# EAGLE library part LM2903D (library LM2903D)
LM2903DG4, Dual Comparator Open Collector 1.3s 2-kanalers 3, 5, 9, 12, 15, 18, 24, 28V 8-Pin SOIC Source: Datasheet
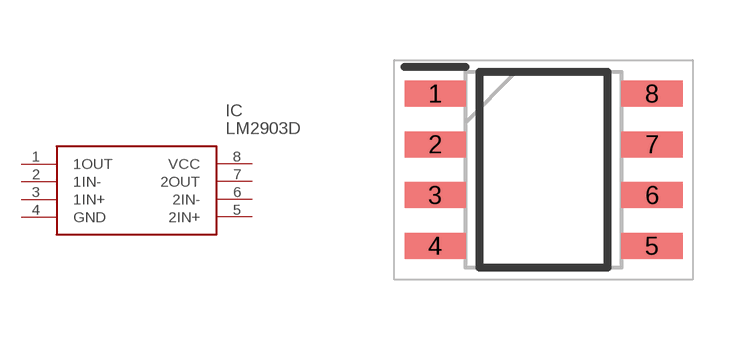
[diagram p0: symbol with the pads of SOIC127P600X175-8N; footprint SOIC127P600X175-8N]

Designator prefix IC

## LM2903D (Arrow_Part_Number: LM2903D; Arrow_Price-Stock: https://www.arrow.com/en/products/lm2903d/texas-instruments; Description: LM2903DG4, Dual Comparator Open Collector 1.3s 2-kanalers 3, 5, 9, 12, 15, 18, 24, 28V 8-Pin SOIC; Height: 1.75mm; Manufacturer_Name: Texas Instruments; Manufacturer_Part_Number: LM2903D; Mouser_Part_Number: 595-LM2903D; Mouser_Price-Stock: https://www.mouser.co.uk/ProductDetail/Texas-Instruments/LM2903D?qs=3pnr37ZAbK86ajtOsfWBBw%3D%3D)  [SOIC127P600X175-8N]
1  1OUT
2  1IN-
3  1IN+
4  GND
5  2IN+
6  2IN-
7  2OUT
8  VCC

## Footprint SOIC127P600X175-8N (pad centres in mm)
+soic d
smd 1.528 x 0.65: 1 -2.711,1.905; 2 -2.711,0.635; 3 -2.711,-0.635; 4 -2.711,-1.905; 5 2.711,-1.905; 6 2.711,-0.635; 7 2.711,0.635; 8 2.711,1.905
